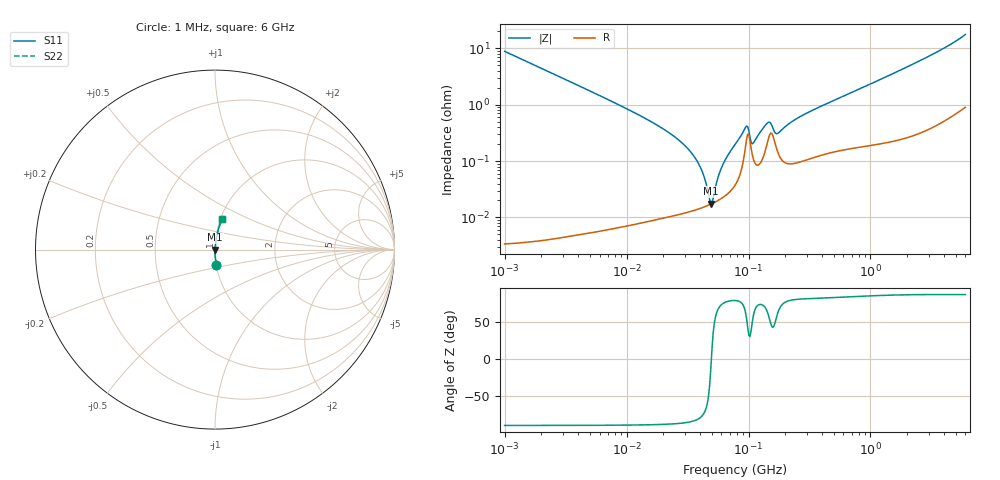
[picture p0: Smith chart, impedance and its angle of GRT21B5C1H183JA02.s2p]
!Murata Part Number: GRT21B5C1H183JA02
!These Parameters are Measured in Series Mode Connection
!Data Generated on Jun 19, 2026
!  o--ll--o
!Port1  Port2
!  o------o
!Operation Temp=25[degC], DC Bias Voltage=0[V]
!Freq. Start=1000[kHz] Stop=6[GHz] 401[Steps]
# Hz S RI R 50
!Freq.(Hz) S11(Real) S11(Imag) S21(Real) S21(Imag) S12(Real) S12(Imag) S22(Real) S22(Imag)
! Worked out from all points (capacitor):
!   401 points, 1 MHz to 6 GHz, reference 50 ohm
!   read as one part in series: C = 17.9 nF near 1.044 MHz
!   lowest |Z| = 17.7 mohm at 49.06 MHz (marker M1)
!   series resonance near 49.59 MHz, so ESL is about 580 pH
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1000000  0.00789 -0.0883  0.9921 0.0883  0.9921 0.0883  0.00789 -0.0883
4293785  0.000472 -0.0205  0.9995 0.0205  0.9995 0.0205  0.000472 -0.0205
1.843659e7  0.000111 -0.00416  0.9999 0.00416  0.9999 0.00416  0.000111 -0.00416
2.727078e7  0.000119 -0.00228  0.9999 0.00228  0.9999 0.00228  0.000119 -0.00228
3.540316e7  0.000134 -0.00125  0.9999 0.00125  0.9999 0.00125  0.000134 -0.00125
4.12249e7  0.000148 -0.000678  0.9999 0.000678  0.9999 0.000678  0.000148 -0.000678
4.905945e7  0.000172 -3.96e-05  0.9998 3.96e-05  0.9998 3.96e-05  0.000172 -3.96e-05
5.124051e7  0.00018 0.000122  0.9998 -0.000122  0.9998 -0.000122  0.00018 0.000122
5.589783e7  0.000199 0.000452  0.9998 -0.000452  0.9998 -0.000452  0.000199 0.000452
6.097846e7  0.000223 0.000795  0.9998 -0.000795  0.9998 -0.000795  0.000223 0.000795
7.745967e7  0.000375 0.00192  0.9996 -0.00192  0.9996 -0.00192  0.000375 0.00192
9.420718e7  0.00173 0.00351  0.9983 -0.00351  0.9983 -0.00351  0.00173 0.00351
9.83954e7  0.00301 0.00278  0.997 -0.00278  0.997 -0.00278  0.00301 0.00278
1.050294e8  0.00169 0.00134  0.9983 -0.00134  0.9983 -0.00134  0.00169 0.00134
1.096987e8  0.00108 0.0018  0.9989 -0.0018  0.9989 -0.0018  0.00108 0.0018
1.424119e8  0.00209 0.00423  0.9979 -0.00423  0.9979 -0.00423  0.00209 0.00423
1.487431e8  0.00291 0.00394  0.9971 -0.00394  0.9971 -0.00394  0.00291 0.00394
1.732027e8  0.00147 0.00272  0.9985 -0.00272  0.9985 -0.00272  0.00147 0.00272
2.297971e8  0.000923 0.00503  0.9991 -0.00503  0.9991 -0.00503  0.000923 0.00503
3.325952e8  0.00119 0.00783  0.9988 -0.00783  0.9988 -0.00783  0.00119 0.00783
1.428092e9  0.00327 0.0331  0.9967 -0.0331  0.9967 -0.0331  0.00327 0.0331
6e9  0.0385 0.1685  0.9615 -0.1685  0.9615 -0.1685  0.0385 0.1685
